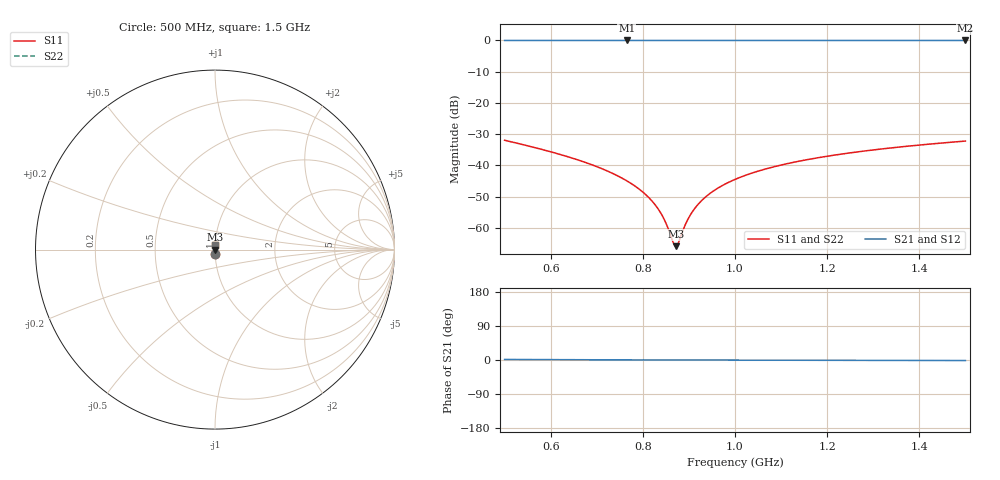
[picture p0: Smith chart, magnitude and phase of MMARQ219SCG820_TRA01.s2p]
! MMARQ219SCG820_TRA01  S-PARAMETER MODEL  ( General Type )
! Model Generated by TAIYO YUDEN Corporation (http://www.ty-top.com)
! Version 1.0
! TAIYO YUDEN Control No. 180601
! Copyright(c) 2018 TAIYO YUDEN CO.,LTD. All Rights Reserved.
! Product Description (link to TY-COMPAS)
! https://ds.yuden.co.jp/TYCOMPAS/or/detail?pn=MMARQ219SCG820JTRA01&u=M
! Products Name : Multilayer Ceramic Capacitors
! Characteristics :
!  Capacitance : 82 pF , Rated Voltage : 250V , TCC : CG / C0G
!  Case Size : 2.0 x 1.25 / 0.079 x 0.049 [mm/inch] , Thickness : 0.85 / 0.033 [mm/inch]
!  (Conditions: Temperature = 25 degC , DC Bias Current/Voltage = 0A / 0V)
! External Node Assignments :
!  1  o---| |---o  2
! GND o---------o GND
! Frequency Range : 500MHz  -  1500MHz  [ 401 STEP ]
# MHz S RI R 50
! Freq[MHz].  S11 Real  S11 Imag  S21 Real  S21 Imag  S12 Real  S12 Imag  S22 Real  S22 Imag
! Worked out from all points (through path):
!   401 points, 500 MHz to 1.5 GHz, reference 50 ohm
!   highest |S21| = 0.00 dB at 765 MHz (marker M1); lowest = 0.0 dB at 1.5 GHz (marker M2)
!   lowest |S11| = -65.9 dB at 872.5 MHz (marker M3), VSWR 1.00, Z = 50.1 + j0.00397 ohm
!   |S11| at or under -10 dB: start of sweep to end of sweep
!   |S22| runs from -65.9 to -31.9 dB; largest |S21 - S12| = 0
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500  0.00104 -0.0253  0.999 0.0253  0.999 0.0253  0.00104 -0.0253
592.5  0.000713 -0.0171  0.9993 0.0171  0.9993 0.0171  0.000713 -0.0171
667.5  0.000577 -0.0117  0.9994 0.0117  0.9994 0.0117  0.000577 -0.0117
722.5  0.000524 -0.00815  0.9995 0.00815  0.9995 0.00815  0.000524 -0.00815
765  0.000503 -0.00565  0.9995 0.00565  0.9995 0.00565  0.000503 -0.00565
805  0.000497 -0.00344  0.9995 0.00344  0.9995 0.00344  0.000497 -0.00344
822.5  0.000497 -0.00251  0.9995 0.00251  0.9995 0.00251  0.000497 -0.00251
835  0.000498 -0.00186  0.9995 0.00186  0.9995 0.00186  0.000498 -0.00186
850  0.000501 -0.00109  0.9995 0.00109  0.9995 0.00109  0.000501 -0.00109
865  0.000506 -0.000333  0.9995 0.000333  0.9995 0.000333  0.000506 -0.000333
870  0.000507 -8.42e-05  0.9995 8.42e-05  0.9995 8.42e-05  0.000507 -8.42e-05
872.5  0.000508 3.96e-05  0.9995 -3.96e-05  0.9995 -3.96e-05  0.000508 3.96e-05
877.5  0.00051 0.000286  0.9995 -0.000286  0.9995 -0.000286  0.00051 0.000286
890  0.000516 0.000896  0.9995 -0.000896  0.9995 -0.000896  0.000516 0.000896
900  0.00052 0.00138  0.9995 -0.00138  0.9995 -0.00138  0.00052 0.00138
920  0.000531 0.00233  0.9995 -0.00233  0.9995 -0.00233  0.000531 0.00233
955  0.000555 0.00394  0.9994 -0.00394  0.9994 -0.00394  0.000555 0.00394
1000  0.000592 0.00594  0.9994 -0.00594  0.9994 -0.00594  0.000592 0.00594
1072.5  0.000667 0.009  0.9993 -0.009  0.9993 -0.009  0.000667 0.009
1167.5  0.00079 0.0128  0.9992 -0.0128  0.9992 -0.0128  0.00079 0.0128
1335  0.00106 0.0189  0.9989 -0.0189  0.9989 -0.0189  0.00106 0.0189
1500  0.00138 0.0245  0.9986 -0.0245  0.9986 -0.0245  0.00138 0.0245
